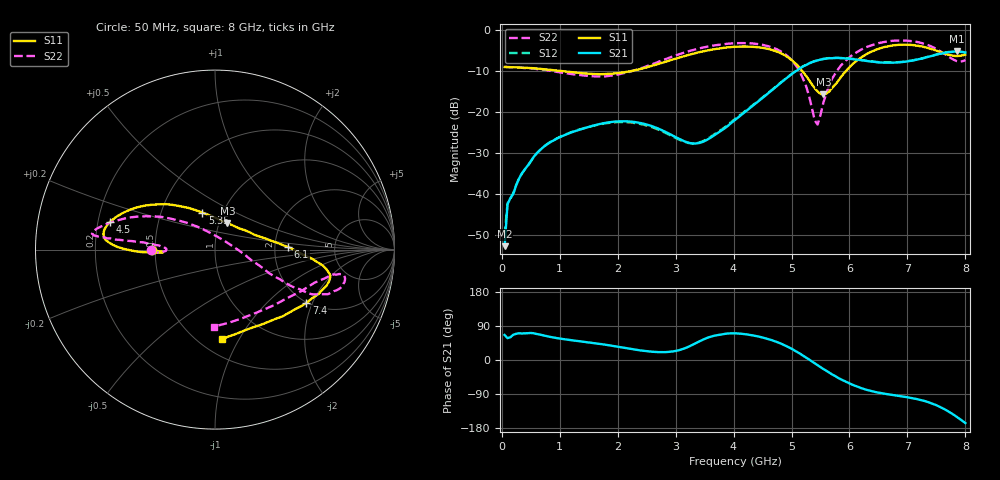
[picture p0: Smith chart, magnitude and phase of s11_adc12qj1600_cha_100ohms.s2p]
#  HZ  S  DB  R  100.00
! Rohde & Schwarz ZVA24 4Ports - Version 4.10 - 1145.1110k26 SN: 100644
! Date: 2020-07-21 15:12:19
! Measurements: S11 S31 S13 S33
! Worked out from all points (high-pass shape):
!   160 points, 50 MHz to 8 GHz, reference 100 ohm
!   highest |S21| = -5.26 dB at 7.85 GHz (marker M1); lowest = -52.7 dB at 50 MHz (marker M2)
!   |S21| within 3 dB of the highest: 5.291 GHz to end of sweep
!   lowest |S11| = -15.7 dB at 5.55 GHz (marker M3), VSWR 1.39, Z = 109 + j33.3 ohm
!   |S11| at or under -10 dB: 1.01 GHz to 2.246 GHz (1.235 GHz wide, 75.9 % of centre); 5.182 GHz to 5.941 GHz (758.8 MHz wide, 13.6 % of centre)
!   |S22| runs from -23.1 to -2.6 dB; largest |S21 - S12| = 0.0042
!   S11 on the Smith chart (normalised r, x): 50 MHz: 0.48, -0.00; 4.5 GHz: 0.25, +0.12; 5.35 GHz: 0.80, +0.35; 6.1 GHz: 2.38, +0.08; 7.4 GHz: 1.98, -1.81; 8 GHz: 0.64, -0.85
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5e7  -9.04 -179.6  -52.74 66.1  -50.04 37.7  -8.98 -179.9
1e8  -9.08 179.8  -42.53 57.6  -42.25 56.7  -9.05 -179.8
3.5e8  -9.20 -179.3  -34.96 70.1  -34.97 70.6  -9.24 -178.2
8e8  -9.67 -178.7  -27.75 62.2  -27.65 62.3  -9.88 -177.1
1.4e9  -10.57 -177.9  -24.07 48.2  -24.03 47.3  -11.07 -178.2
2.1e9  -10.36 -176.8  -22.28 32.4  -22.49 31.8  -10.55 176.7
2.7e9  -8.31 -177.7  -24.05 20.9  -24.32 21.7  -7.79 174.2
3.4e9  -5.45 178.8  -27.61 48.3  -27.49 51.0  -4.52 174.0
4.05e9  -4.09 173.1  -21.65 70.4  -21.45 70.4  -3.23 172.7
4.5e9  -4.37 165.2  -16.60 59.4  -16.47 59.2  -3.63 169.3
5.05e9  -7.97 140.8  -10.26 25.4  -10.21 25.2  -8.21 151.5
5.25e9  -11.17 122.7  -8.58 6.6  -8.52 6.5  -13.65 135.1
5.35e9  -13.22 108.8  -7.89 -3.6  -7.84 -3.8  -18.90 114.2
5.45e9  -15.00 89.5  -7.44 -13.6  -7.38 -13.8  -23.09 49.6
5.55e9  -15.74 65.1  -7.10 -23.8  -7.06 -24.0  -17.72 -1.1
5.75e9  -13.40 27.3  -6.86 -42.1  -6.80 -42.4  -10.76 -21.4
6.1e9  -7.78 2.0  -7.17 -68.1  -7.12 -68.4  -5.64 -25.0
6.7e9  -3.91 -10.6  -8.00 -91.4  -7.94 -91.7  -2.71 -16.9
7.05e9  -3.65 -16.6  -7.55 -99.7  -7.50 -100.0  -2.69 -11.4
7.4e9  -4.59 -30.3  -6.42 -113.6  -6.38 -113.8  -3.96 -14.5
7.85e9  -6.38 -69.1  -5.26 -149.8  -5.23 -150.1  -7.60 -59.2
8e9  -6.02 -85.6  -5.51 -166.4  -5.48 -166.8  -7.36 -90.5
